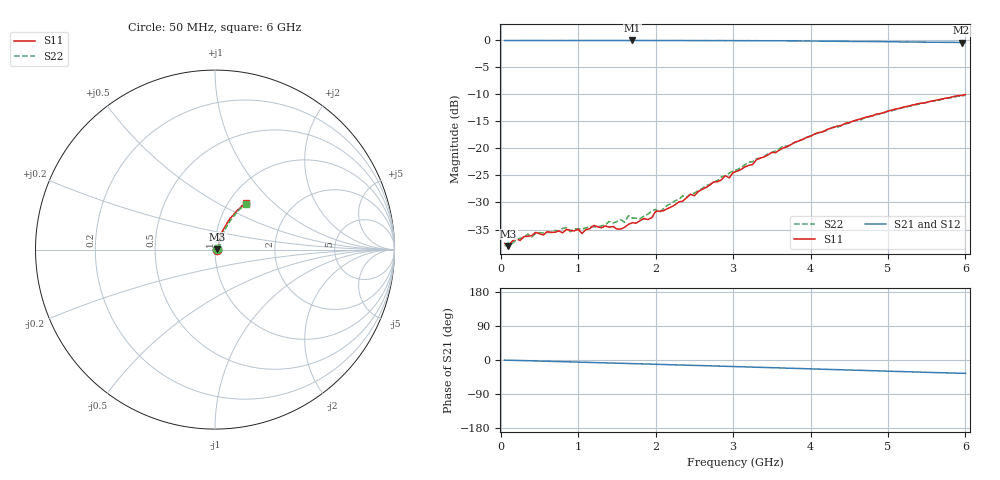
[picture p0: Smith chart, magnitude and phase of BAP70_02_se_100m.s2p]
!	Created	by	janssen	on	Thu	Dec	12	13:21:17	MET	2002
#	HZ	S	MA	R	50
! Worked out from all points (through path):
!   120 points, 50 MHz to 6 GHz, reference 50 ohm
!   highest |S21| = -0.09 dB at 1.7 GHz (marker M1); lowest = -0.5 dB at 5.95 GHz (marker M2)
!   group delay of S21, straight-line fit = 16.6 ps
!   lowest |S11| = -38.0 dB at 100 MHz (marker M3), VSWR 1.03, Z = 51.3 + j0.0733 ohm
!   |S11| at or under -10 dB: start of sweep to end of sweep
!   |S22| runs from -38.1 to -10.2 dB; largest |S21 - S12| = 0.0081
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5e7  0.01324 2.1  0.9885 -0.4  0.9872 -0.5  0.01249 2.9
1e8  0.01257 3.3  0.9877 -0.6  0.9873 -0.6  0.01348 3.4
2e8  0.01463 8.0  0.9879 -1.1  0.9879 -1.2  0.01424 10.0
2.5e8  0.0141 4.3  0.988 -1.4  0.9878 -1.4  0.01478 4.5
4.5e8  0.01675 4.8  0.9885 -2.5  0.9878 -2.5  0.01635 4.2
5.5e8  0.01586 9.5  0.9886 -3.0  0.9884 -3.1  0.01656 5.5
1e9  0.01789 5.0  0.9882 -5.5  0.9884 -5.7  0.01801 1.3
1.05e9  0.01635 6.0  0.9889 -5.8  0.9883 -5.8  0.01797 4.3
1.2e9  0.01942 9.3  0.9885 -6.7  0.9875 -6.7  0.01881 6.7
1.55e9  0.018 18.7  0.9885 -8.7  0.9872 -8.7  0.02187 16.0
1.7e9  0.02057 25.6  0.9894 -9.5  0.9878 -9.6  0.02269 26.0
1.8e9  0.02146 28.6  0.9888 -10.1  0.988 -10.2  0.02233 23.5
1.95e9  0.02283 36.5  0.9878 -11.0  0.9881 -11.0  0.02636 27.7
2e9  0.0261 39.1  0.9877 -11.3  0.9877 -11.4  0.02728 34.7
2.05e9  0.02632 41.1  0.988 -11.6  0.9877 -11.6  0.02562 34.5
2.35e9  0.03253 52.8  0.9882 -13.3  0.9873 -13.4  0.03644 43.5
2.4e9  0.03491 52.8  0.9869 -13.7  0.9868 -13.7  0.03523 44.6
3.05e9  0.06141 63.4  0.985 -17.5  0.9846 -17.4  0.0631 57.5
4.05e9  0.1351 66.9  0.9769 -23.7  0.9761 -23.5  0.1351 63.2
5.05e9  0.2253 62.1  0.9624 -29.9  0.9646 -29.6  0.2217 59.9
5.95e9  0.3074 56.1  0.9466 -35.0  0.954 -34.9  0.3034 56.2
6e9  0.3134 56.2  0.9475 -35.2  0.9523 -35.2  0.3087 56.1
